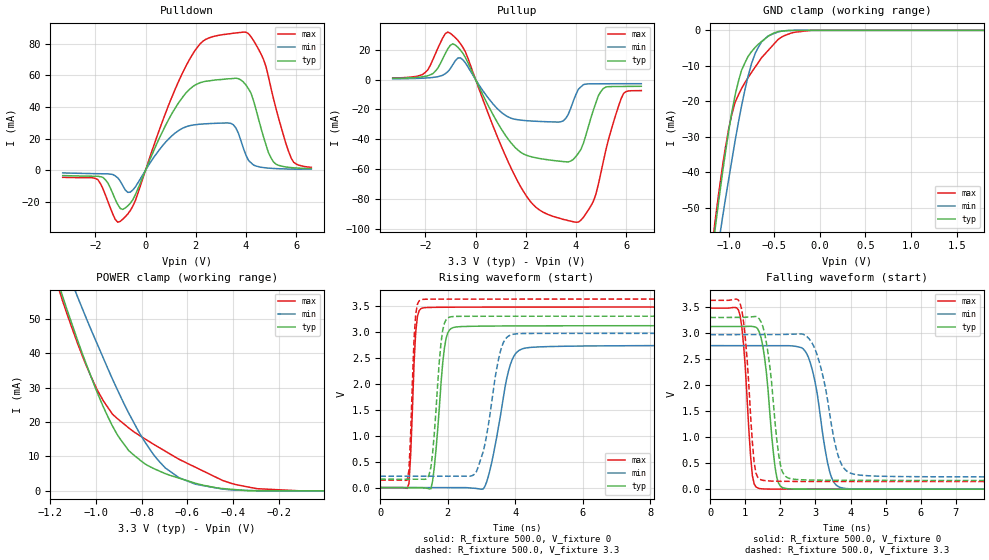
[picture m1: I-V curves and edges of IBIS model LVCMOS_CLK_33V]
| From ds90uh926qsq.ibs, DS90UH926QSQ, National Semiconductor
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[Model] LVCMOS_CLK_33V
Model_type 3-state
Enable Active-High
Vmeas = 1.65V
Cref = 0.0pF
Rref = 1.0e10
Vref = 0.0V
C_comp   2.75pF   2.32pF   3.18pF
[Voltage Range]   3.3V   2.98V   3.63V
[Temperature Range]   25.0   130.0   -40.0
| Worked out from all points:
|   slope of the pulldown table from 0 to 0.495 V, typ, clamps not added: 26.8 ohm
|   slope of the pullup table from 0 to 0.495 V, typ, clamps not added: 28.9 ohm
|   GND clamp passes 1 mA (typ) near -0.52 V on its own axis
|   POWER clamp passes 1 mA (typ) near -0.48 V on its own axis
|   rising waveform, R_fixture 500.0, V_fixture 0: 20-80 % time 231ps typ, 459ps min, 129ps max; typ from 0 V to 3.12 V
|   falling waveform, R_fixture 500.0, V_fixture 0: 20-80 % time 259ps typ, 393ps min, 196ps max; typ from 3.13 V to 0 V
|   rising waveform, R_fixture 500.0, V_fixture 3.3: 20-80 % time 216ps typ, 411ps min, 122ps max; typ from 0.162 V to 3.3 V
|   falling waveform, R_fixture 500.0, V_fixture 3.3: 20-80 % time 293ps typ, 475ps min, 214ps max; typ from 3.3 V to 0.166 V
[GND Clamp]
-1.792V   -197.8mA   -186.4mA   -214.7mA
-1.149V   -56.47mA   -67.17mA   -54.23mA
-1.069V   -40.73mA   -53.29mA   -38.77mA
-968.2mV  -23.71mA   -37.34mA   -24.18mA
-928mV    -18.23mA   -31.14mA   -20.29mA
-857.7mV  -11.28mA   -21.35mA   -16.43mA
-787.3mV  -7.409mA   -13.09mA   -13.4mA
-706.9mV  -4.766mA   -6.44mA    -10.3mA
-566.2mV  -1.656mA   -1.584mA   -5.676mA
-385.3mV  -149.1uA   -109.1uA   -1.469mA
-93.81mV  -1.103uA   -8.052uA   -4.704uA
1.796V    990.9nA    0A         -3.355uA
[POWER Clamp]
-1.792V   198mA      187.8mA    214.3mA
-1.169V   61.3mA     71.7mA     60.11mA
-1.149V   57.22mA    68.23mA    55.84mA
-1.079V   43.45mA    56.1mA     42.54mA
-988.3mV  27.6mA     41.74mA    28.59mA
-897.9mV  15.44mA    28.2mA     20.54mA
-857.7mV  11.77mA    22.72mA    18.35mA
-787.3mV  7.898mA    14.35mA    15.17mA
-696.9mV  5.007mA    6.677mA    11.54mA
-566.2mV  2.233mA    1.97mA     6.902mA
-385.3mV  327.7uA    202.5uA    1.779mA
-3.35mV   3.487uA    -7.649uA   -8.998uA
[Pullup]
-3.3V     799.7uA    508.1uA    1.021mA
-2.104V   1.84mA     892.9uA    3.394mA
-1.008V   22.86mA    7.19mA     30.95mA
-606.4mV  19.73mA    14.48mA    24.06mA
891.2mV   -29.35mA   -19.87mA   -39.23mA
1.997V    -50.45mA   -27.47mA   -77.18mA
3.494V    -54.86mA   -27.59mA   -93.52mA
3.997V    -51.4mA    -9.927mA   -95.37mA
4.69V     -20.49mA   -2.871mA   -81.41mA
5.092V    -5.936mA   -2.841mA   -54.35mA
5.896V    -4.625mA   -2.807mA   -9.253mA
6.6V      -4.537mA   -2.795mA   -7.404mA
[Pulldown]
-3.3V     -3.479mA   -1.778mA   -4.581mA
-1.903V   -3.912mA   -2.276mA   -5.98mA
-1.008V   -24.29mA   -6.98mA    -32.51mA
-606.4mV  -20.93mA   -13.94mA   -25.58mA
891.2mV   31.27mA    19.31mA    40.1mA
1.896V    53.11mA    28.58mA    74.01mA
3.394V    57.9mA     29.6mA     86.49mA
3.896V    55.79mA    13.78mA    87.45mA
4.69V     21.38mA    1.617mA    70.34mA
5.092V    5.212mA    1.044mA    45.32mA
5.796V    1.588mA    643.4uA    7.7mA
6.6V      989.9uA    600.4uA    1.724mA
[Rising Waveform]
R_fixture=500.0
V_fixture=0
V_fixture_min=0
V_fixture_max=0
0s        25.57nV    547.7nV    68.32nV
850ps     -3.124uV   553.1nV    79.97mV
1.05ns    2.218uV    549.4nV    2.999V
1.3ns     -6.06mV    538nV      3.463V
1.95ns    2.876V     -4.352uV   3.473V
2.25ns    3.093V     6.122uV    3.474V
3.1ns     3.11V      24.79mV    3.475V
3.85ns    3.113V     2.363V     3.476V
4.45ns    3.114V     2.7V       3.476V
49.98ns   3.12V      2.746V     3.478V
[Falling Waveform]
R_fixture=500.0
V_fixture=0
V_fixture_min=0
V_fixture_max=0
0s        3.126V     2.759V     3.48V
850ps     3.126V     2.759V     3.341V
1.2ns     3.128V     2.759V     264.8mV
1.45ns    2.909V     2.759V     8.22mV
1.9ns     216.6mV    2.759V     901uV
2.2ns     8.808mV    2.759V     551.4uV
2.8ns     900.2uV    2.532V     225.1uV
3.4ns     378.3uV    348.9mV    99.53uV
3.9ns     209.4uV    10.22mV    75.96uV
49.98ns   5.158uV    13.88uV    2.983uV
[Rising Waveform]
R_fixture=500.0
V_fixture=3.3
V_fixture_min=2.97
V_fixture_max=3.63
0s        162.1mV    218.4mV    144.5mV
800ps     162.1mV    218.4mV    146.2mV
1.05ns    162.1mV    218.4mV    3.339V
1.25ns    160.7mV    218.4mV    3.623V
1.5ns     392.5mV    218.4mV    3.628V
1.85ns    3.034V     218.4mV    3.629V
2.15ns    3.293V     218.4mV    3.629V
2.85ns    3.299V     310.7mV    3.63V
4.05ns    3.3V       2.962V     3.63V
49.98ns   3.3V       2.97V      3.63V
[Falling Waveform]
R_fixture=500.0
V_fixture=3.3
V_fixture_min=2.97
V_fixture_max=3.63
0s        3.3V       2.97V      3.63V
850ps     3.301V     2.97V      3.571V
1.25ns    3.317V     2.97V      520.2mV
1.6ns     2.819V     2.97V      161mV
2ns       467.4mV    2.972V     151mV
2.45ns    187.2mV    2.982V     148.2mV
3.05ns    172.8mV    2.576V     146.9mV
3.75ns    169.1mV    467.4mV    146.5mV
4.3ns     168.3mV    267.4mV    146.4mV
49.98ns   165.5mV    228.6mV    145.7mV
[Ramp]
R_load = 500.0
dV/dt_r   1.872108E0/2.5E-10   1.647706E0/4.5E-10   2.086516E0/1E-10
dV/dt_f   1.880685E0/3E-10   1.64484E0/4.5E-10   2.090601E0/2.5E-10
